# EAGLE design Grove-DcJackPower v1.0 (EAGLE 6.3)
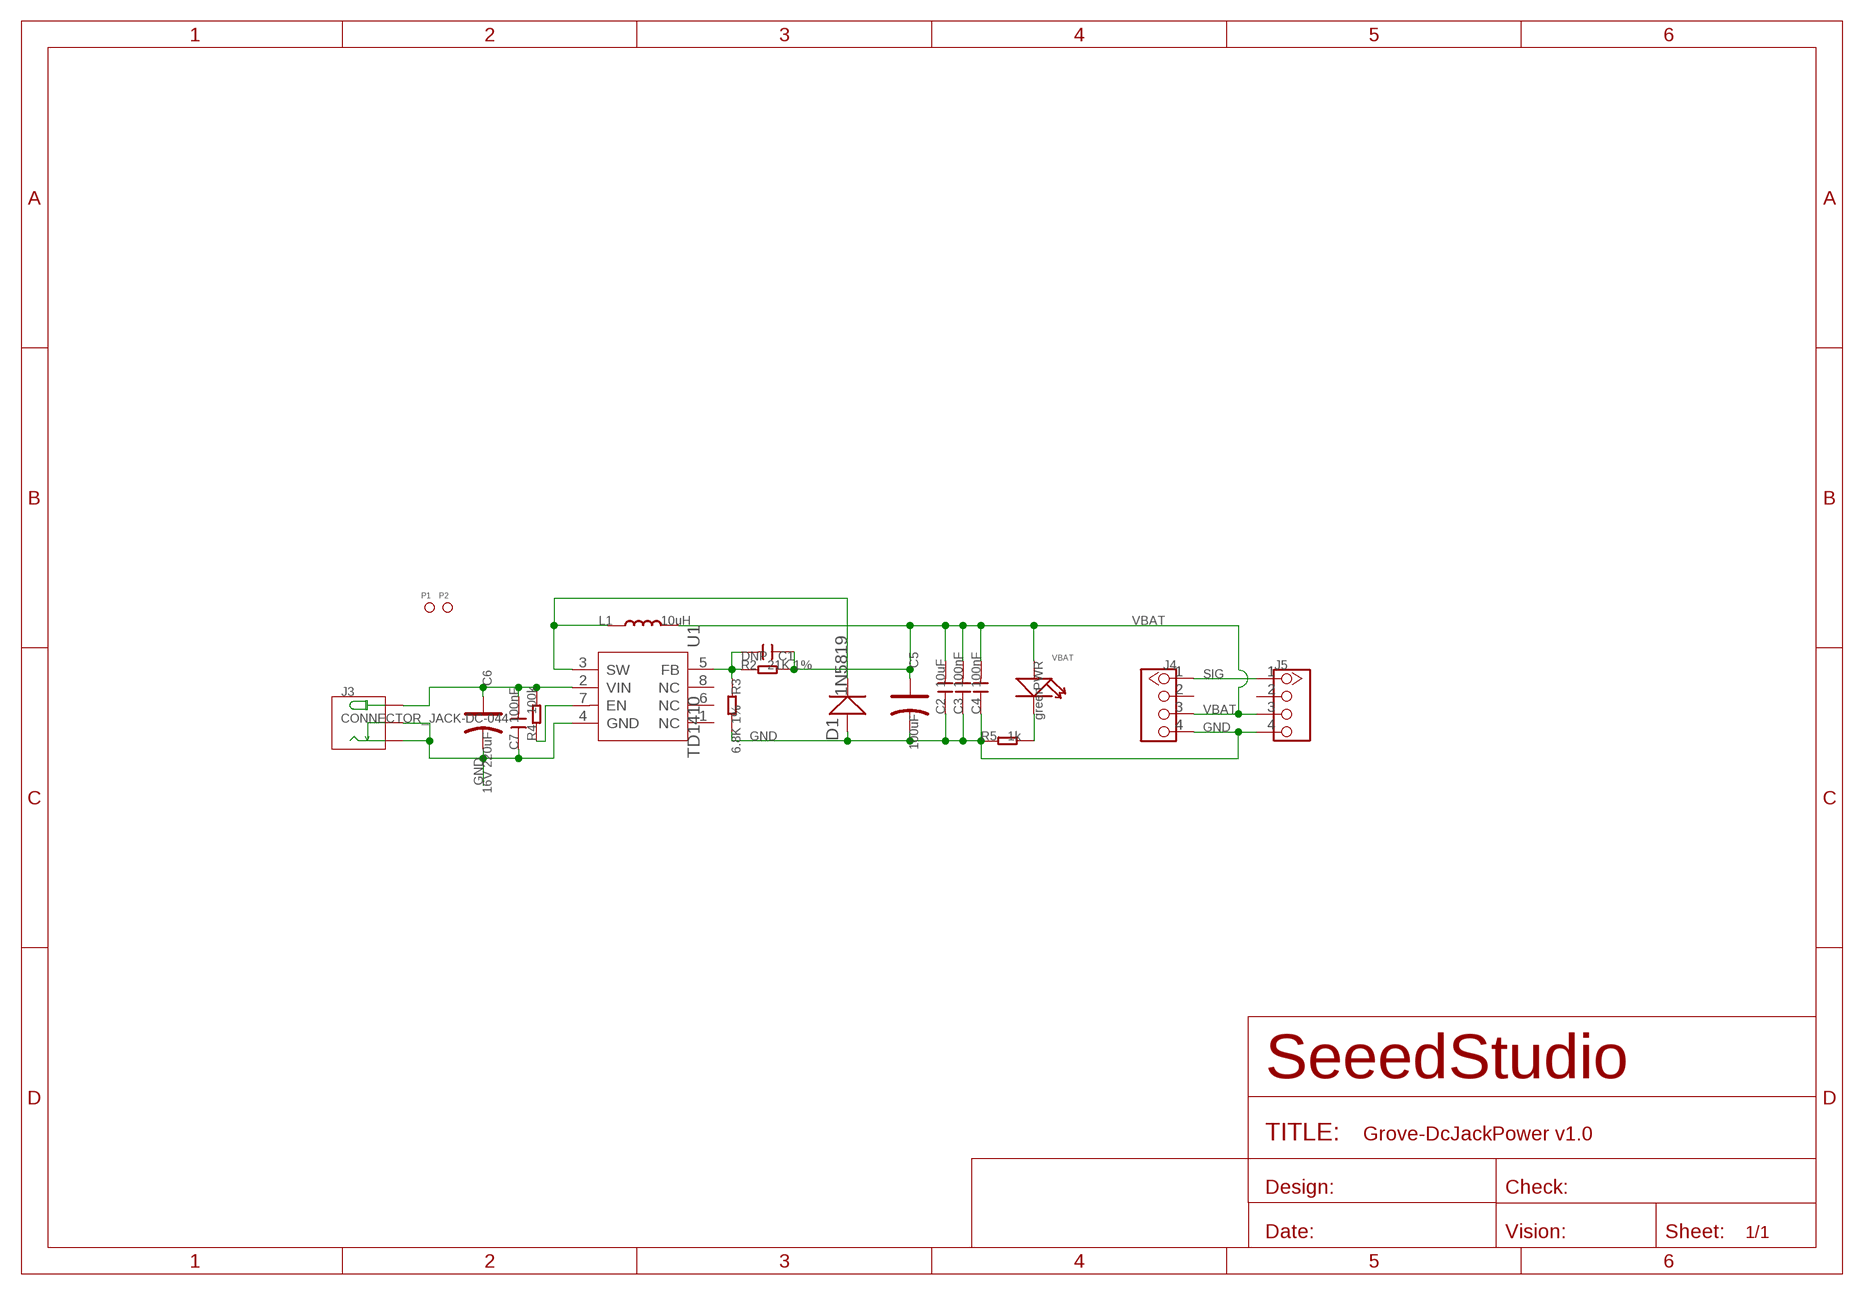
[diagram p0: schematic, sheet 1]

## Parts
C1  DNP  C-0603  [C0603]
C2  10uF  C-0805  [C0805]
C3  100nF  C-0603  [C0603]
C4  100nF  C-0603  [C0603]
C5  100uF  CAP-AVX-B  [AVX-B]
C6  16V 220uF  CAP-ELECTRO-D  [ELECTRO-SMD-D-5.6MM]
C7  100nF  C-0603  [C0603]
D1  1N5819  D'SMA'  [D2010]
J3  CONNECTOR_JACK-DC-044  [CONNECTOR_DC-404]
J4  TWIG-4P-2.0'90D'  [4P-2.0-90D]
J5  TWIG-4P-2.0'90D'  [4P-2.0-90D]
L1  10uH  L'0630'  [L0630]
P1  PAD-MARK  [ROUND-MARK-1.0]
P2  PAD-MARK  [ROUND-MARK-1.0]
PWR  green  007-LED0603  [D0603]
R2  21K 1%  R-0603  [R0603]
R3  6.8K 1%  R-0603  [R0603]
R4  100k  R-0603  [R0603]
R5  1k  R-0603  [R0603]
U1  TD1410  [SOP8]

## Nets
GND: C2.1 C3.1 C4.1 C5.- C6.- C7.1 D1.+ J3.- J3.CDN J4.4 J5.4 R3.2 R5.1 U1.4(GND)
N$1: PWR.- R5.2
N$52: R4.1 U1.7(EN)
N$53: D1.- L1.1 U1.3(SW)
N$54: C1.2 R2.1 R3.1 U1.5(FB)
SIG: J4.1 J5.1
VBAT: C1.1 C2.2 C3.2 C4.2 C5.+ J4.3 J5.3 L1.2 PWR.+ R2.2
VIN: C6.+ C7.2 J3.+ R4.2 U1.2(VIN)
Unconnected: J4.2 J5.2 U1.1(NC) U1.6(NC) U1.8(NC)

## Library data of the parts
C1-C4 C7 = Discrete:C*: Ceramic Capacitors
C5 C6 = Discrete:CAP*: Electrolytic Capacitors,Tantalum Capacitors and Super Capacitors
D1 = Discrete:D*
J3 = Grove-DcJackPower:CONNECTOR_JACK-DC-044
J4 J5 = Connector:TWIG-4P-2.0
L1 = Discrete:L*
P1 P2 = Discrete:PAD-MARK; PARTNO: DNP
PWR = Discrete:007-LED*
R2-R5 = Discrete:R*
U1 = template:TD1410: 2A 380KHz 20V PWM Buck DC/DC Converter

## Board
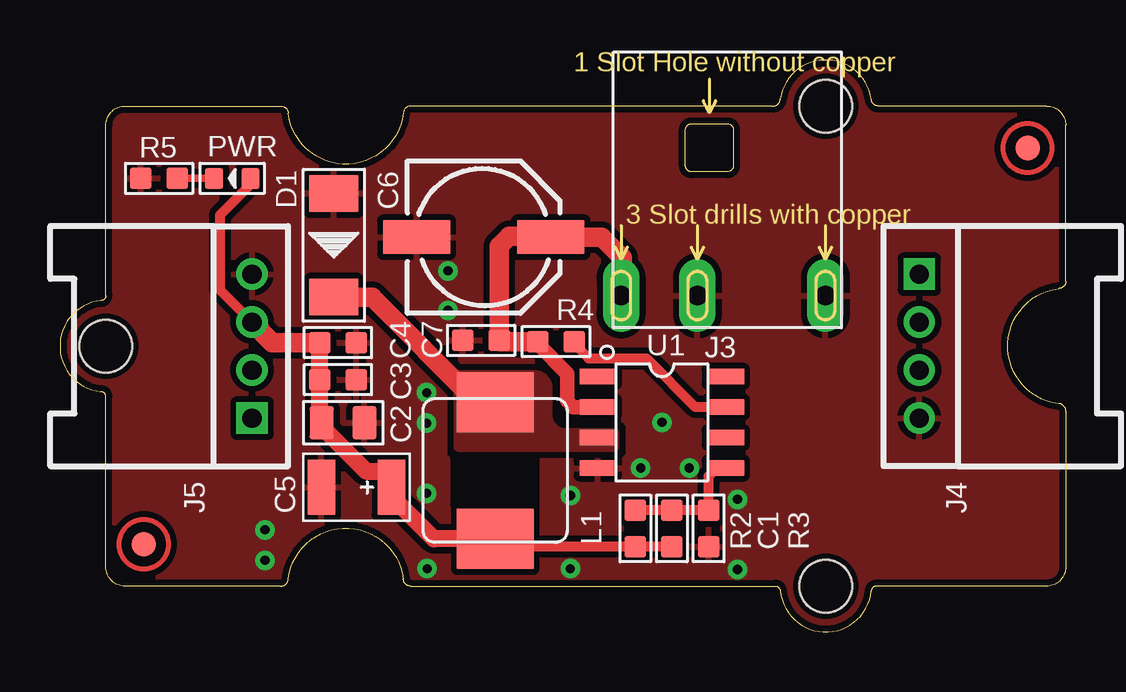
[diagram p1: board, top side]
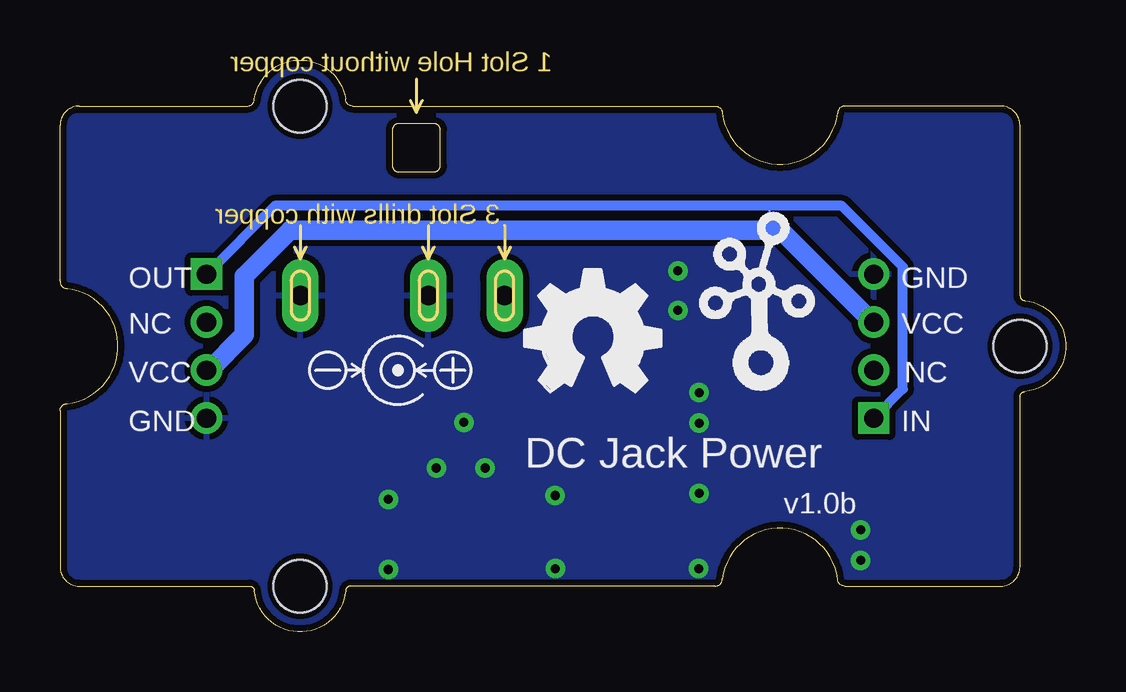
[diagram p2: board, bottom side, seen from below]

Size 41.91 x 23.83 mm. Coordinates in mm from the lower left corner, seen from the top.
Copper layers (1*16): Top 0.035mm / dielectric 1.5mm / Bottom 0.035mm
Design rules "default *": minimum track width 8mil, minimum drill 12mil, track to track 8mil, track to pad 8mil, pad to pad 8mil, via to via 8mil, smd to smd 0mil, copper to edge 10mil, drill to drill 8mil, minimum pad ring 10mil, minimum via ring 8mil, stop-mask expansion 4mil, vias tented up to drill 25mil, thermal gap 10mil
tRestrict: area 16.5,5.3 to 19.7,7.2

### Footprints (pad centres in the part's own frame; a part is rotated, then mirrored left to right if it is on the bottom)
C0603 = smd 0.889 x 0.889: 1 -0.762,0; 2 0.762,0
C0805 = smd 1.016 x 1.397: 1 -0.889,0; 2 0.889,0
AVX-B = smd 1.143 x 2.286: + -1.46,0; - 1.46,0
ELECTRO-SMD-D-5.6MM = smd 2.794 x 1.397: + 2.794,0; - -2.794,0
D2010 = smd 1.524 x 2.032: + -2.159,0; - 2.159,0
CONNECTOR_DC-404 = drill 0.813 pad 1.524 long: + 3.175,10.16; - -5.334,10.16; CDN 0,10.16
4P-2.0-90D = drill 0.8 pad 1.27 square: 1 -3,0 | drill 0.8 pad 1.27: 2 -1,0; 3 1,0; 4 3,0
L0630 = smd 2.5 x 3.2: 1 -2.85,0; 2 2.85,0
ROUND-MARK-1.0 = smd 1.016 x 1.016: P$1 0,0
D0603 = smd 0.762 x 0.889: + -0.762,0; - 0.762,0
R0603 = smd 0.889 x 0.889: 1 -0.762,0; 2 0.762,0
SOP8 = smd 0.635 x 1.524: 1 -1.905,-2.667; 2 -0.635,-2.667; 3 0.635,-2.667; 4 1.905,-2.667; 5 1.905,2.667; 6 0.635,2.667; 7 -0.635,2.667; 8 -1.905,2.667
2U-DIM-W/DRILL = hole 2.2: -10,-10; -10,10; 20,0

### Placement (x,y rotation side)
C1  25.5,4.32 90 top
C2  11.8,8.71 180 top
C3  11.58,10.51 180 top
C4  11.58,12.06 180 top
C5  12.35,6.02 180 top
C6  17.65,16.45 0 top
C7  17.55,12.14 0 top
D1  11.41,16.11 270 top
J3  26.56,24.17 180 top
J4  35.8,11.91 270 top
J5  8,11.91 90 top
L1  18.13,6.73 270 top
P1  3.49,3.65 0 top
P2  40.32,20.16 0 top
PWR  7.18,18.89 180 top
R2  23.98,4.32 270 top
R3  27.02,4.32 270 top
R4  20.67,12.1 180 top
R5  4.13,18.89 0 top
U1  25.08,8.73 270 top
U$2  [2U-DIM-W/DRILL]  21.91,11.91 0 bottom
U$3  [OSHW_FILLX200_NOTEXT]  22.54,10 0 bottom
U$4  [TWIGLOGO]  12.76,11.02 0 bottom

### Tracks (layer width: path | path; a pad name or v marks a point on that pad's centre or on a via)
GND  (via drill 0.38 pad 0.81)
  other vias: 21.27,2.64 15.3,2.64 28.23,2.6 24.19,6.83 26.23,6.83 25.08,8.73 28.23,5.52 15.28,9.97 15.28,8.7 8.54,2.98 8.54,4.25 15.28,5.78 16.16,13.4 16.16,15.05 21.27,5.69
  pour Bottom (isolate 0.254, rank 2): -0.32,-0.16 42.22,-0.16 42.22,23.97 -0.32,23.97 -0.32,-0.03
  pour Top (isolate 0.254, rank 2): -0.32,-0.16 42.22,-0.16 42.22,23.97 -0.32,23.97 -0.32,-0.03
N$1
  Top 0.305: PWR.- R5.2
N$52
  Top 0.406: R4.1 21.43,12 22.03,11.4 24.44,11.4 26.47,9.37 U1.7
N$53
  Top 0.813: L1.1 17.37,9.58 13.01,13.94 D1.-
  pour Top (isolate 0.254, no thermals): 16.61,7.62 23.09,7.62 arc90 23.21,7.74 23.21,8.25 arc90 23.09,8.38 21.05,8.38 arc-90 20.42,9.01 20.42,10.16 arc90 19.78,10.79 16.61,10.79 arc90 16.48,10.67 16.48,7.74 arc90
N$54
  Top 0.406: R2.1 C1.2 R3.1 27.02,6.49 27.36,6.83 U1.5
SIG
  Bottom 0.406: J5.1 6.79,10.12 6.79,15.21 9.33,17.75 32.96,17.75 J4.1
VBAT
  Top 0.406: C1.1 R2.2 18.46,3.55 L1.2 | PWR.+ 7.94,18.64 6.66,17.37 6.66,14.25 J5.3
  Top 0.711: C2.2 10.91,8.55 12.76,6.7 13.9,6.7 13.9,6.12 C5.+ 13.81,5.65 15.58,3.88 L1.2 | 10.82,8.81 C3.2 C4.2
  Top 0.813: C4.2 8.85,12.06 J5.3 | 10.82,8.81 C2.2
  Bottom 0.813: J5.3 8.04,12.91 11.87,16.73 32.32,16.73 34.22,14.83 34.22,12.37 35.69,10.91 J4.3
VIN
  Top 0.61: R4.2 19.9,12 21.14,10.77 21.14,9.62 21.39,9.37 U1.2
  Top 0.813: J3.+ 23.43,14.06 23.43,15.59 22.57,16.45 C6.+ 20.42,16.48 18.73,16.48 18.31,16.06 C7.2 18.36,12.1 R4.2

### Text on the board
bPlace: GND | OUT | VCC | NC | NC | VCC | IN | GND | DC Jack Power | v1.0b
